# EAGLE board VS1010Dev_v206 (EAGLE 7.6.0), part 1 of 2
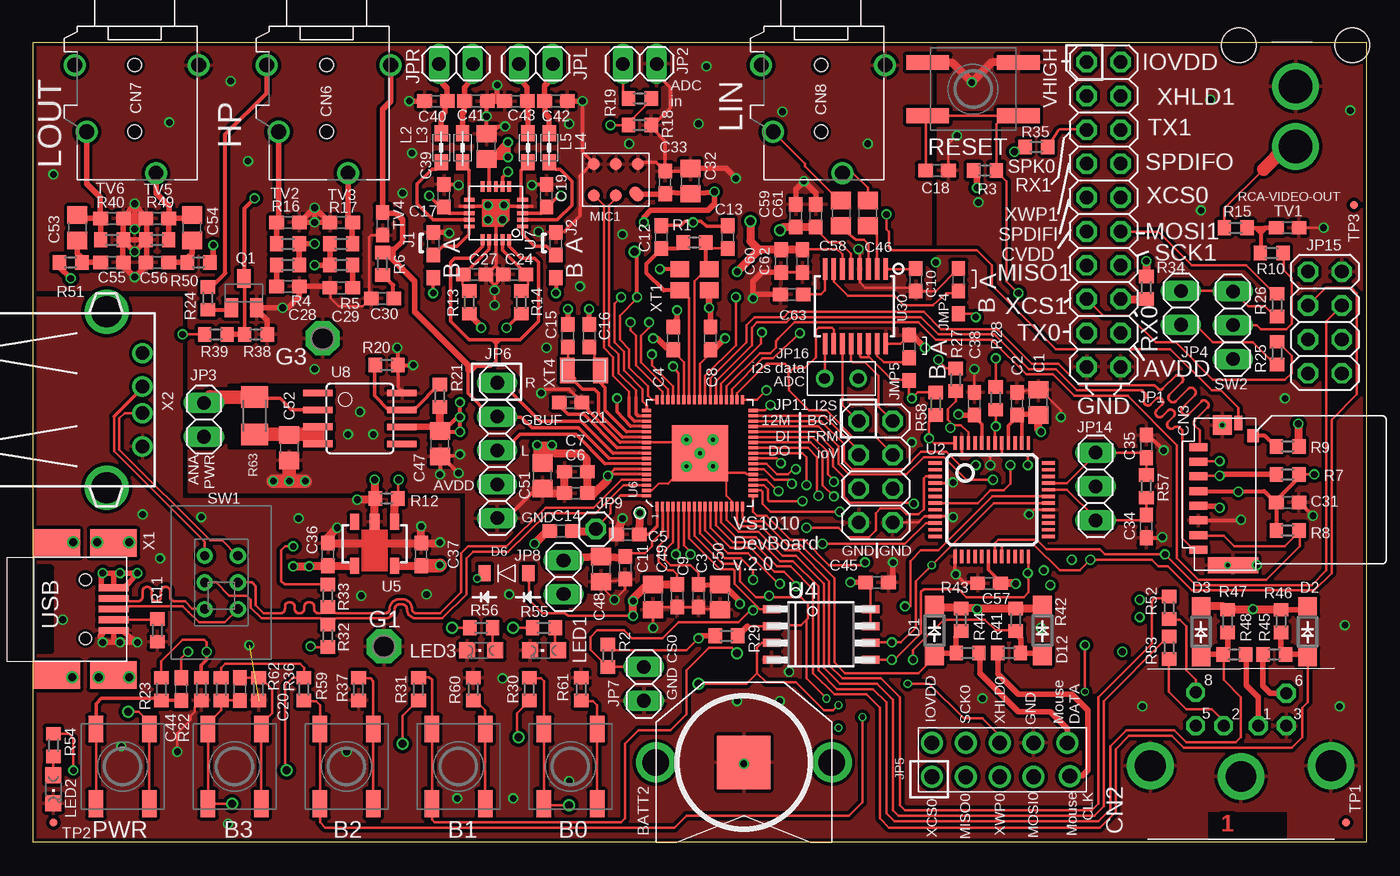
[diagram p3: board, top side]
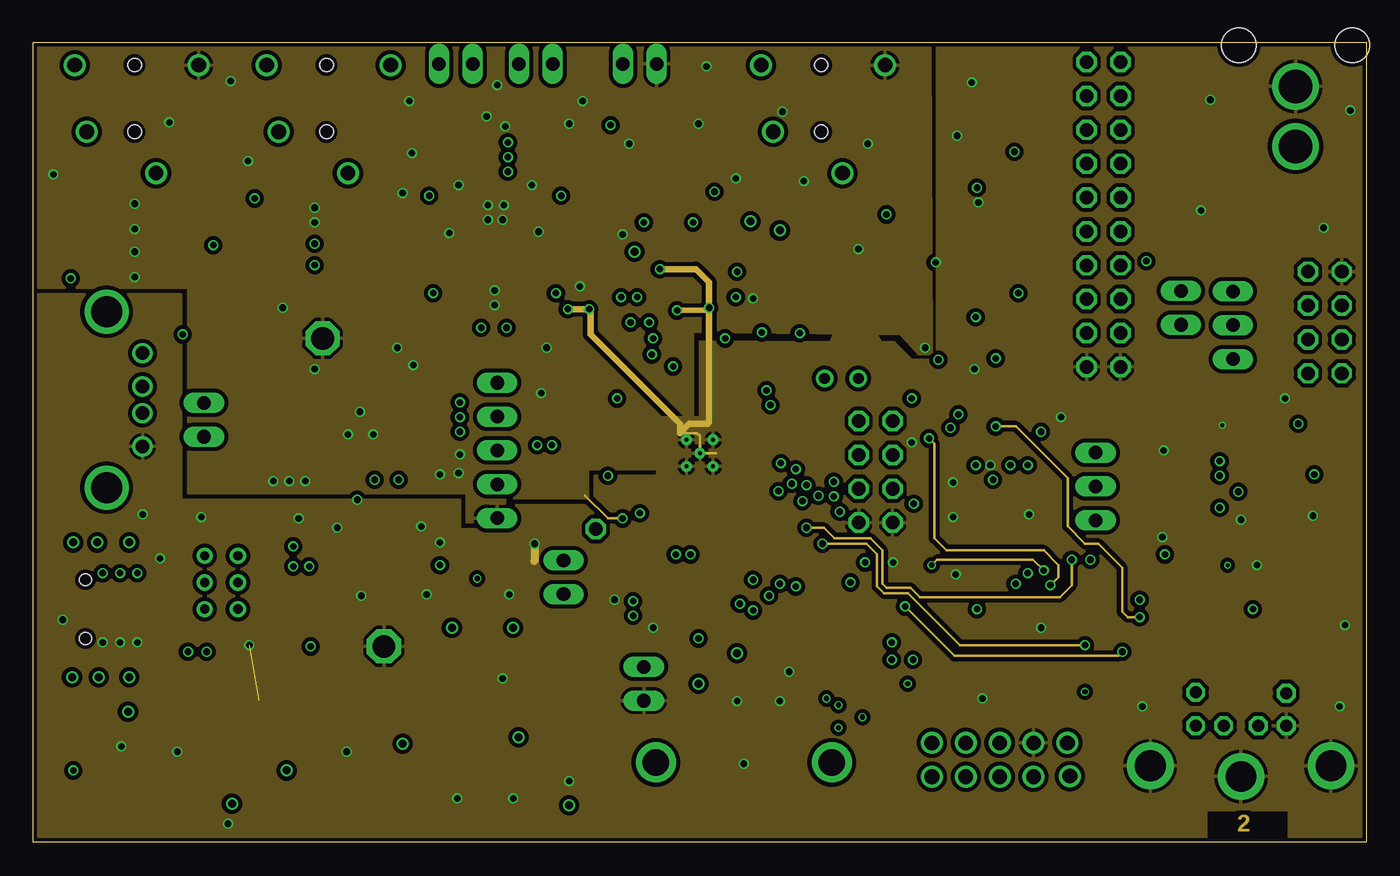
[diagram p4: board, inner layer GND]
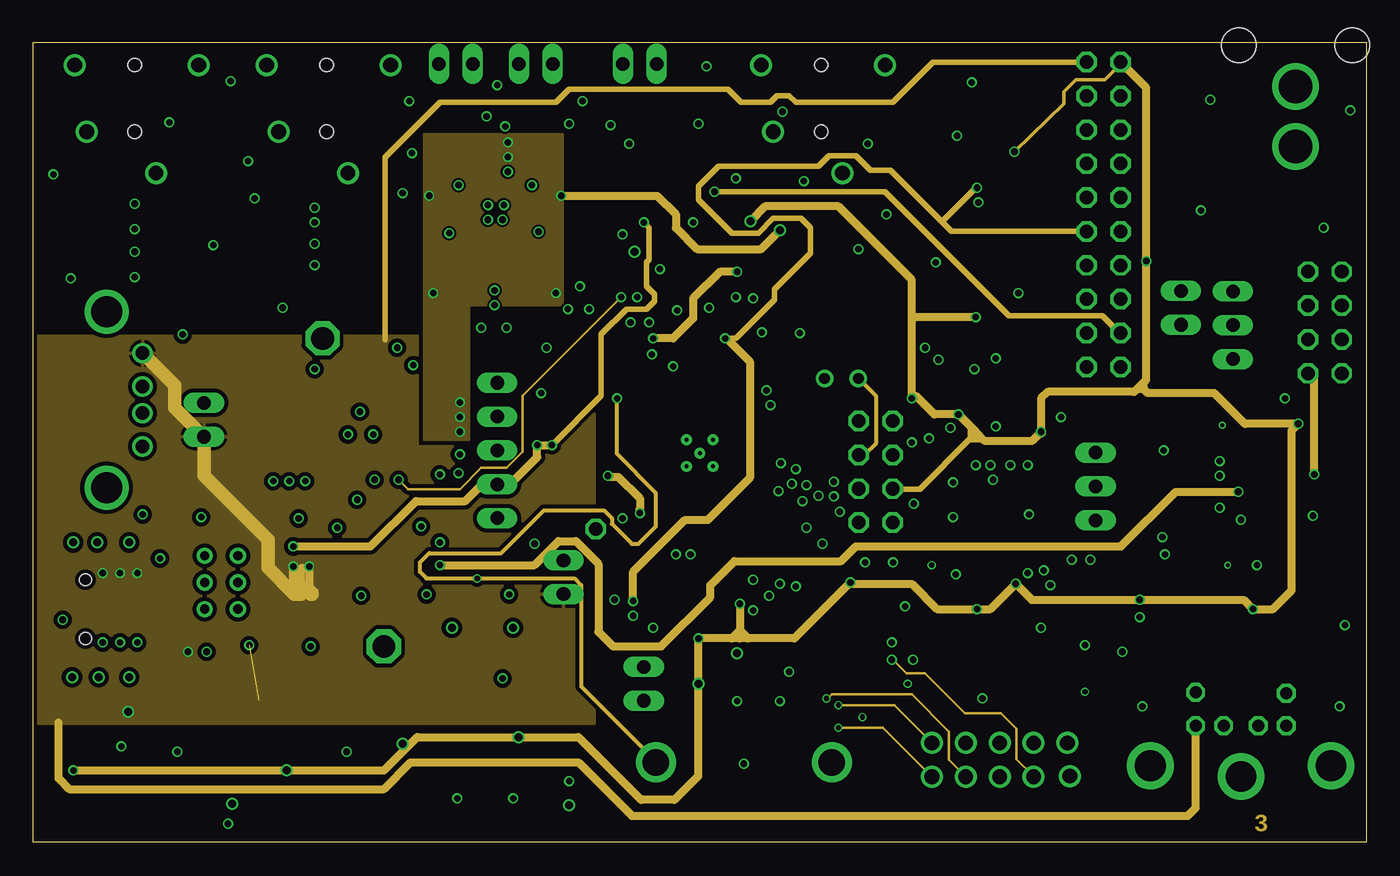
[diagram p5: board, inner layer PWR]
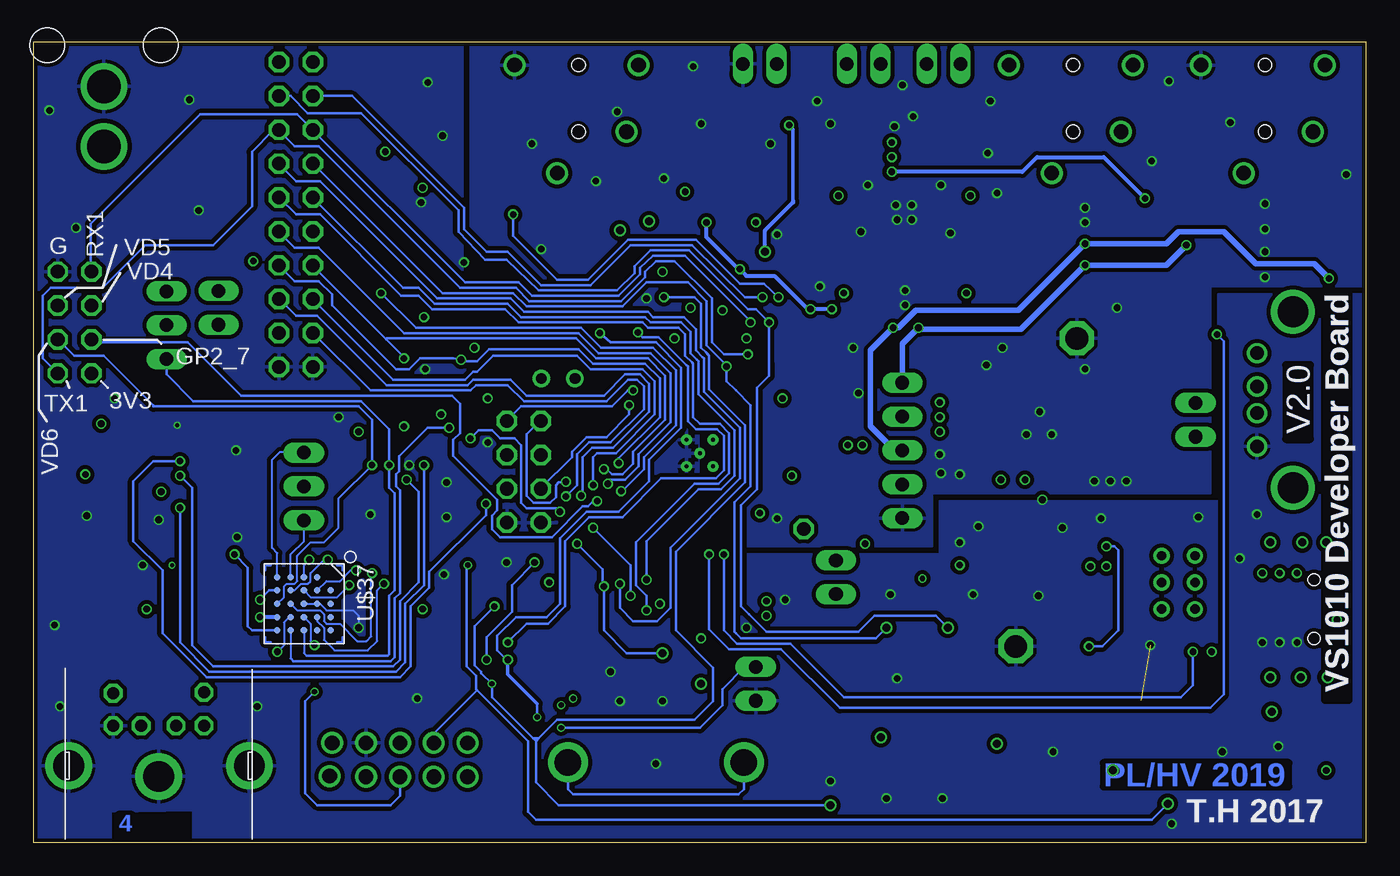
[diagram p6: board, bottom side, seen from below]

Size 100 x 60 mm. Coordinates in mm from the lower left corner, seen from the top.
Outline: 100,0 0,0 0,60 100,60 100,0
Copper layers ((1*2+3*16)): Top 0.035mm / dielectric 0.12mm / GND 0.0175mm / dielectric 1.2mm / PWR 0.035mm / dielectric 0.2mm / Bottom 0.035mm
Design rules "4L_Smart_prototyping_Eagle Rule *": minimum track width 6mil, minimum drill 0.3mm, track to track 6mil, track to pad 6mil, pad to pad 6mil, via to via 6mil, smd to smd 0mil, copper to edge 6mil, drill to drill 12mil, minimum pad ring 10mil, minimum via ring 4mil, stop-mask expansion 2mil, vias tented up to drill 25mil, thermal gap 10mil
tRestrict: area 48.5,25.6 to 53.6,32.8; area 33.1,45.6 to 36.3,48.8

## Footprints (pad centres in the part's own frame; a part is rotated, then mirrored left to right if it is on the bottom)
SW_EVQ_MINI = smd 2 x 1.1: A -2.8,2; A1 2.8,2; B -2.8,-2; B1 2.8,-2
KS2997 = smd 4 x 4: NEG 0,0 | drill 2: P1 -6.6,0; P2 6.6,0
C0805 = smd 1.3 x 1.5: 1 -0.95,0; 2 0.95,0
C0603 = smd 1.1 x 1: 1 -0.85,0; 2 0.85,0
M_DIN6 = drill 0.9 pad 1.422 octagon: 1 -1.3,-3.75; 2 1.3,-3.75; 3 -3.4,-3.75; 5 3.4,-3.75; 6 -3.4,-6.2; 8 3.4,-6.25 | drill 2.3 pad 3.5: SH1 6.8,-0.75; SH2 0,0.05; SH3 -6.75,-0.75
MSSN09-A0-3000 = smd 0.6 x 1.35: 1 3.85,0.1; 2 2.75,0.1; 3 1.65,0.1; 4 0.55,0.1; 5 -0.55,0.1; 6 -1.65,0.1; 7 -2.75,0.1; 8 -3.85,0.1 | smd 1.2 x 3.79: 9 -5,-2.5 | smd 1.45 x 1.4: 10 5.5,-1.7 | smd 1.1 x 0.6: 11 5.65,-2.9 | smd 0.95 x 0.85: 12 4.7,-4
SJ-43514 = drill 1.1: 1 8.1,1.6; 4 5,-3.6; 5 0,4.8; 6 0,-4.5 | hole 1: 0,0; 5,0
SOD123 = smd 1.4 x 1.4: A 1.9,0; C -1.9,0
SOD-123 = smd 0.914 x 1.219: ANODE -1.638,0; CATHODE 1.638,0
P1-17 = drill 1.702 pad 2.54 octagon: TP 0,0
0603X2 = smd 1.1 x 1: 1 -0.85,0; 2 0.85,0; 3 2.55,0
2X10 = drill 1.016 octagon: 1 -11.43,-1.27; 2 -11.43,1.27; 3 -8.89,-1.27; 4 -8.89,1.27; 5 -6.35,-1.27; 6 -6.35,1.27; 7 -3.81,-1.27; 8 -3.81,1.27; 9 -1.27,-1.27; 10 -1.27,1.27; 11 1.27,-1.27; 12 1.27,1.27; 13 3.81,-1.27; 14 3.81,1.27; 15 6.35,-1.27; 16 6.35,1.27; 17 8.89,-1.27; 18 8.89,1.27; 19 11.43,-1.27; 20 11.43,1.27
1X02 = drill 1.016 long: 1 -1.27,0; 2 1.27,0
2X5_2.54MM_CON = drill 1.1: 1 -5.08,-1.27; 2 -5.08,1.27; 3 -2.54,-1.27; 4 -2.54,1.27; 5 0,-1.27; 6 0,1.27; 7 2.54,-1.27; 8 2.54,1.27; 9 5.27,-1.22; 10 5.08,1.27
1X05 = drill 1.016 long: 1 -5.08,0; 2 -2.54,0; 3 0,0; 4 2.54,0; 5 5.08,0
1X01 = drill 1.016 octagon: 1 0,0
2X04 = drill 1.016 octagon: 1 -3.81,-1.27; 2 -3.81,1.27; 3 -1.27,-1.27; 4 -1.27,1.27; 5 1.27,-1.27; 6 1.27,1.27; 7 3.81,-1.27; 8 3.81,1.27
1X03 = drill 1.016 long: 1 -2.54,0; 2 0,0; 3 2.54,0
2X1_2.54MM_CON_THROUGH = drill 0.8: P$1 0,0; P$2 2.54,0
0805 = smd 1.2 x 1: 1 -1.1,0; 2 1.1,0
CHIPLED_0805 = smd 1.2 x 1.2: A 0,-1.05; C 0,1.05
MIC_MEMS_CMM-4737DT = smd 0.91 x 0.91: 1 -1.17,1.65; 2 -1.17,0; 3 -1.17,-1.65; 4 1.17,-1.65; 5 1.17,0 | smd 1.2 x 0.91 rotated 45: 6 1.07,1.55
SOT23-BEC = smd 1 x 1.4: B -0.95,-1.1; C 0,1.1; E 0.95,-1.1
R0603 = smd 1 x 1.1: 1 -0.85,0; 2 0.85,0
M1206 = smd 1.6 x 2: 1 -1.4,0; 2 1.4,0
1X1_RCA_CON_RCJ-044 = drill 2.5: 1 -4,0; 2 -8.5,0 | hole 2.6: -0.9,4.25; -0.9,-4.25
SW_EVQ = smd 3.2 x 1.1: A -3.4,2; A1 3.4,2; B -3.4,-2; B1 3.4,-2
SW_ALPS_SSSS922500 = drill 0.7: 1 -2,-1.25; 2 0,-1.25; 3 2,-1.25; 4 -2,1.25; 5 0,1.25; 6 2,1.25
TP06R = smd 0.6 x 0.6: TP 0,0
0603 = smd 1.1 x 1: 1 -0.85,0; 2 0.85,0
LQFP48 = smd 0.25 x 1: 1 -2.75,-4.25; 2 -2.25,-4.25; 3 -1.75,-4.25; 4 -1.25,-4.25; 5 -0.75,-4.25; 6 -0.25,-4.25; 7 0.25,-4.25; 8 0.75,-4.25; 9 1.25,-4.25; 10 1.75,-4.25; 11 2.25,-4.25; 12 2.75,-4.25; 25 2.75,4.25; 26 2.25,4.25; 27 1.75,4.25; 28 1.25,4.25; 29 0.75,4.25; 30 0.25,4.25; 31 -0.25,4.25; 32 -0.75,4.25; 33 -1.25,4.25; 34 -1.75,4.25; 35 -2.25,4.25; 36 -2.75,4.25 | smd 1 x 0.25: 13 4.25,-2.75; 14 4.25,-2.25; 15 4.25,-1.75; 16 4.25,-1.25; 17 4.25,-0.75; 18 4.25,-0.25; 19 4.25,0.25; 20 4.25,0.75; 21 4.25,1.25; 22 4.25,1.75; 23 4.25,2.25; 24 4.25,2.75; 37 -4.25,2.75; 38 -4.25,2.25; 39 -4.25,1.75; 40 -4.25,1.25; 41 -4.25,0.75; 42 -4.25,0.25; 43 -4.25,-0.25; 44 -4.25,-0.75; 45 -4.25,-1.25; 46 -4.25,-1.75; 47 -4.25,-2.25; 48 -4.25,-2.75
SO8-SHORT = smd 1.3 x 0.6: 1 -3.913,1.905; 2 -3.913,0.635; 3 -3.913,-0.635; 4 -3.913,-1.905; 5 3.513,-1.905; 6 3.513,-0.635; 7 3.513,0.635; 8 3.513,1.905
SOT89-5 = smd 0.68 x 1.2: 1 -1.5,-1.65; 3 1.5,-1.65; 4 1.5,1.65; 5 -1.5,1.65 | smd 0.76 x 1.2: 2 0,-1.65
QFN68 = smd 0.7 x 0.23: 1 -4,3.2; 2 -4,2.8; 3 -4,2.4; 4 -4,2; 5 -4,1.6; 6 -4,1.2; 7 -4,0.8; 8 -4,0.4; 9 -4,0; 10 -4,-0.4; 11 -4,-0.8; 12 -4,-1.2; 13 -4,-1.6; 14 -4,-2; 15 -4,-2.4; 16 -4,-2.8; 17 -4,-3.2; 35 4,-3.2; 36 4,-2.8; 37 4,-2.4; 38 4,-2; 39 4,-1.6; 40 4,-1.2; 41 4,-0.8; 42 4,-0.4; 43 4,0; 44 4,0.4; 45 4,0.8; 46 4,1.2; 47 4,1.6; 48 4,2; 49 4,2.4; 50 4,2.8; 51 4,3.2 | smd 0.23 x 0.7: 18 -3.2,-4; 19 -2.8,-4; 20 -2.4,-4; 21 -2,-4; 22 -1.6,-4; 23 -1.2,-4; 24 -0.8,-4; 25 -0.4,-4; 26 0,-4; 27 0.4,-4; 28 0.8,-4; 29 1.2,-4; 30 1.6,-4; 31 2,-4; 32 2.4,-4; 33 2.8,-4; 34 3.2,-4; 52 3.2,4; 53 2.8,4; 54 2.4,4; 55 2,4; 56 1.6,4; 57 1.2,4; 58 0.8,4; 59 0.4,4; 60 0,4; 61 -0.4,4; 62 -0.8,4; 63 -1.2,4; 64 -1.6,4; 65 -2,4; 66 -2.4,4; 67 -2.8,4; 68 -3.2,4 | smd 4.2 x 4.2: GNDPAD 0,0 | drill 0.3: P$1 -1,1; P$2 1,1; P$3 1,-1; P$4 -1,-1; P$5 0,0
QFN20 = smd 0.8 x 0.28: 1 -2,1; 2 -2,0.5; 3 -2,0; 4 -2,-0.5; 5 -2,-1; 11 2,-1; 12 2,-0.5; 13 2,0; 14 2,0.5; 15 2,1 | smd 0.28 x 0.8: 6 -1,-2; 7 -0.5,-2; 8 0,-2; 9 0.5,-2; 10 1,-2; 16 1,2; 17 0.5,2; 18 0,2; 19 -0.5,2; 20 -1,2
SOIC8 = smd 0.5 x 2.2: 1 -1.905,-3.354; 2 -0.645,-3.354; 3 0.625,-3.354; 4 1.895,-3.354; 5 1.905,2.954; 6 0.635,2.954; 7 -0.635,2.954; 8 -1.905,2.954
TSSOP16 = smd 1.6 x 0.35: 1 -2.9,2.45; 2 -2.9,1.8; 3 -2.9,1.15; 4 -2.9,0.5; 5 -2.9,-0.15; 6 -2.9,-0.8; 7 -2.9,-1.45; 8 -2.9,-2.1; 9 2.7,-2.1; 10 2.7,-1.45; 11 2.7,-0.8; 12 2.7,-0.15; 13 2.7,0.5; 14 2.7,1.15; 15 2.7,1.8; 16 2.7,2.45
BGA24_5X5 = smd 0.5 x 0.5: A2 1,0; A3 2,0; A4 3,0; A5 4,0; B1 0,-1; B2 1,-1; B3 2,-1; B4 3,-1; B5 4,-1; C1 0,-2; C2 1,-2; C3 2,-2; C4 3,-2; C5 4,-2; D1 0,-3; D2 1,-3; D3 2,-3; D4 3,-3; D5 4,-3; E1 0,-4; E2 1,-4; E3 2,-4; E4 3,-4; E5 4,-4
MINI_USB_MOLEX-B = smd 2.25 x 0.5: 1 7.915,1.6; 2 7.915,0.8; 3 7.915,0; 4 7.915,-0.8; 5 7.915,-1.6 | smd 3.5 x 2.05: P$6 7.915,4.95; P$7 7.915,-4.95; P$8 3.665,4.95; P$9 3.665,-4.95 | hole 0.9: 5.815,2.2; 5.815,-2.2
USB-S = drill 1: 1 -3.5,12.99; 2 -1,12.99; 3 1,12.99; 4 3.5,12.99 | drill 2.3: P$1 -6.6,10.3; P$2 6.6,10.3
NX3225GA = smd 1.4 x 1.2: 1 -1.1,-0.8; 2 1.1,-0.8; 3 1.1,0.8; 4 -1.1,0.8
CRYSTAL_1206 = smd 1.1 x 1.9: 1 -1.25,0; 2 1.25,0

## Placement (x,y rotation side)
B0  [SW_EVQ_MINI]  40.3,5.7 90 top
B1  [SW_EVQ_MINI]  31.9,5.7 90 top
B2  [SW_EVQ_MINI]  23.5,5.7 90 top
B3  [SW_EVQ_MINI]  15.1,5.7 90 top
BATT2  1.5V LR(SR)44  [KS2997]  53.3,6 180 top
C1  10u  [C0805]  75.4,33 90 top
C2  100n  [C0603]  73.8,32.9 90 top
C3  100n  [C0603]  49.9,18.5 270 top
C4  100n  [C0603]  48,37.8 90 top
C5  100n  [C0603]  44.6,23.1 180 top
C6  100n  [C0603]  40.7,26.2 180 top
C7  100n  [C0603]  40.7,27.8 180 top
C8  100n  [C0603]  50.8,37.8 90 top
C9  100n  [C0603]  48.3,18.5 270 top
C10  470n  [C0603]  66.2,42.2 270 top
C11  100n  [C0603]  44.4,20.6 270 top
C12  4.7p  [C0603]  47.1,45.4 270 top
C13  4.7p  [C0603]  52.1,45.4 270 top
C14  1u  [C0603]  39.59,23.36 180 top
C15  10P  [C0603]  40.1,38 270 top
C16  10P  [C0603]  41.7,38 270 top
C17  100n  [C0603]  30.8,48.5 90 top
C18  1u  [C0603]  67.8,50.4 0 top
C19  100n  [C0603]  38.5,48.5 90 top
C20  100n  [C0603]  15.5,11.5 90 top
C21  1u  [C0603]  40.3,33 0 top
C24  4n7/NP0  [C0603]  36.1,42.6 180 top
C27  4n7/NP0  [C0603]  33.1,42.6 0 top
C28  10n  [C0603]  19.1,41.7 0 top
C29  10n  [C0603]  23.1,41.6 180 top
C30  47n  [C0603]  26.2,40.8 180 top
C31  1u  [C0603]  94.1,25.5 0 top
C32  10u  [C0805]  49.3,49.6 270 top
C33  100n  [C0603]  47.4,49.5 90 top
C34  20P  [C0603]  83.5,23.7 90 top
C35  20P  [C0603]  83.5,29.7 270 top
C36  1u  [C0603]  22.1,21.6 90 top
C37  1u  [C0603]  29.1,21.6 90 top
C38  100n  [C0603]  70.6,32.9 90 top
C39  10u  [C0805]  34,52.2 90 top
C40  1n  [C0603]  30.2,55.6 180 top
C41  1n  [C0603]  33.2,55.6 0 top
C42  1n  [C0603]  39.2,55.6 0 top
C43  1n  [C0603]  36.2,55.6 180 top
C44  dnc  [C0603]  11.1,11.5 90 top
C45  100n  [C0603]  63.3,19.5 0 top
C46  10u  [C0805]  62.6,47.2 270 top
C47  10u  [C0805]  30.5,29.9 90 top
C48  10u  [C0805]  42.6,20.5 270 top
C49  10u  [C0805]  46.5,18.4 270 top
C50  10u  [C0805]  51.5,18.4 270 top
C51  10u  [C0805]  38.2,27.5 270 top
C52  10u  [C0805]  19.2,29.6 270 top
C53  10u  [C0805]  3.3,46.1 90 top
C54  10u  [C0805]  11.9,46.1 90 top
C55  3n3/NP0  [C0603]  5.9,43.5 0 top
C56  3n3/NP0  [C0603]  9.3,43.5 180 top
C57  100n  [C0603]  71.7,19.44 180 top
C58  10u  [C0805]  60.6,47.2 270 top
C59  10u  [C0603]  57.2,47 270 top
C60  10u  [C0603]  56.1,43.6 270 top
C61  100n  [C0603]  58.7,47 270 top
C62  100n  [C0603]  57.7,43.6 270 top
C63  1u  [C0603]  56.9,41.1 180 top
CN2  [M_DIN6]  90.6,5 180 top
CN3  CON-USD-TOMIN  [MSSN09-A0-3000]  87.5,25.8 90 top
CN6  SJ-43514  [SJ-43514]  22,58.3 270 top
CN7  SJ-43514  [SJ-43514]  7.6,58.3 270 top
CN8  SJ-43514  [SJ-43514]  59.1,58.3 270 top
D1  SD103AW  [SOD123]  67.6,15.9 270 top
D2  SD103AW  [SOD123]  95.6,15.8 270 top
D3  SD103AW  [SOD123]  87.6,15.8 270 top
D6  MBR0520  [SOD-123]  35.5,20.2 180 top
D12  SD103AW  [SOD123]  75.7,15.9 270 top
G1  TPPAD1-17  [P1-17]  26.3,14.7 0 top
G3  TPPAD1-17  [P1-17]  21.7,37.8 0 top
J1  100K  [0603X2]  30,44.9 270 top
J2  100K  [0603X2]  39.2,44.9 270 top
JMP4  0R-JMP  [0603X2]  69.4,42.2 270 top
JMP5  0R-JMP  [0603X2]  65.7,37.2 270 top
JP1  [2X10]  80.3,47.1 270 top
JP2  [1X02]  45.5,58.4 180 top
JP3  [1X02]  12.8,31.7 270 top
JP4  [1X02]  86.1,40.1 270 top
JP5  spi0/mouse  [2X5_2.54MM_CON]  72.5,6.2 0 top
JP6  [1X05]  34.8,29.4 270 top
JP7  [1X02]  45.8,11.9 90 top
JP8  [1X02]  39.78,19.89 270 top
JP9  [1X01]  42.2,23.5 0 top
JP11  [2X04]  63.2,27.8 270 top
JP14  SMC-1-03-1-GT  [1X03]  79.7,26.7 270 top
JP15  [2X04]  96.9,39 270 top
JP16  [2X1_2.54MM_CON_THROUGH]  61.9,34.8 180 top
JPL  SPKL  [1X02]  37.7,58.4 180 top
JPR  SPKR  [1X02]  31.7,58.4 0 top
L2  [0805]  30.6,52.1 90 top
L3  [0805]  32.2,52.1 90 top
L4  [0805]  38.7,52.1 90 top
L5  [0805]  37.1,52.1 90 top
LED1  GREEN  [CHIPLED_0805]  38.3,14.4 90 top
LED2  GREEN  [CHIPLED_0805]  1.5,4 180 top
LED3  RED  [CHIPLED_0805]  33.6,14.4 90 top
MIC1  cmm-4737DT-26186-TR  [MIC_MEMS_CMM-4737DT]  43.7,49.7 270 top
PWR  [SW_EVQ_MINI]  6.7,5.7 90 top
Q1  BC850  [SOT23-BEC]  15.8,41.2 0 top
R1  470k  [R0603]  49.6,45 0 top
R2  100k  [R0603]  43.1,14 270 top
R3  100k  [R0603]  71.4,50.4 0 top
R4  20R  [R0603]  19.1,43.3 180 top
R5  20R  [R0603]  23.1,43.3 0 top
R6  10R  [R0603]  26.2,43.4 270 top
R7  11k  [R0603]  94.1,27.6 180 top
R8  11k  [R0603]  94.1,23.4 0 top
R9  11k  [R0603]  94.1,29.7 180 top
R10  22R  [R0603]  92.9,44.2 180 top
R11  100k  [R0603]  9.3,15.9 270 top
R12  100k  [R0603]  26.5,25.8 180 top
R13  1k  [R0603]  32.7,40.5 270 top
R14  1k  [R0603]  36.6,40.5 270 top
R15  22R  [R0603]  90.2,46.1 180 top
R16  10R  [R0603]  19.1,44.9 180 top
R17  10R  [R0603]  23.1,44.9 0 top
R18  2k  [R0603]  45.5,53.8 0 top
R19  18k  [R0603]  45.5,55.8 0 top
R20  11k  [R0603]  26.5,35.8 180 top
R21  51k  [R0603]  30.5,33.5 270 top
R22  100k  [R0603]  12.6,11.5 90 top
R23  51k  [R0603]  9.6,11.5 90 top
R24  100k  [R0603]  13.1,40.8 270 top
R25  100R  [R0603]  93.3,36.7 90 top
R26  100R  [R0603]  93.3,40.3 90 top
R27  11k  [R0603]  69.2,34.7 90 top
R28  11k  [R0603]  72.2,33.3 270 top
R29  100k  [R0603]  52,15.5 0 top
R30  100k  [R0603]  37.2,11.5 270 top
R31  100k  [R0603]  28.9,11.5 270 top
R32  470k  [R0603]  22.1,15.5 90 top
R33  470k  [R0603]  22.1,18.5 270 top
R34  100k  [R0603]  83.5,41.6 90 top
R35  100k  [R0603]  75.25,52.17 180 top
R36  11k  [R0603]  16.9,11.5 270 top
R37  11k  [R0603]  24.4,11.5 270 top
R38  51k  [R0603]  16.7,38.1 0 top
R39  11k  [R0603]  13.7,38.1 0 top
R40  100k  [R0603]  5.9,45.2 0 top
R41  330R  [R0603]  73.2,14.2 0 top
R42  2k  [R0603]  73.7,16.7 270 top
R43  2k  [R0603]  69.6,16.7 270 top
R44  330R  [R0603]  70.1,14.2 0 top
R45  330R  [R0603]  93.1,14.1 180 top
R46  2k  [R0603]  93.6,16.6 270 top
R47  2k  [R0603]  89.6,16.6 270 top
R48  330R  [R0603]  90.1,14.1 180 top
R49  100k  [R0603]  9.3,45.2 180 top
R50  470R  [R0603]  12.4,43.5 180 top
R51  470R  [R0603]  2.8,43.5 0 top
R52  11k  [R0603]  85.2,17.6 90 top
R53  11k  [R0603]  85.2,14.6 90 top
R54  330R  [R0603]  1.5,7.3 270 top
R55  330R  [R0603]  38.3,16.1 0 top
R56  330R  [R0603]  33.6,16.1 0 top
R57  470k  [R0603]  83.5,26.7 270 top
R58  11k  [R0603]  67.7,32.9 270 top
R59  100k  [R0603]  20.3,11.5 90 top
R60  11k  [R0603]  33,11.5 90 top
R61  11k  [R0603]  41.1,11.5 90 top
R62  100k  [R0603]  14.1,11.5 90 top
R63  0  [M1206]  16.6,32 90 top
RCA-VIDEO-OUT  1X1_RCA_CON_RCJ-044  [1X1_RCA_CON_RCJ-044]  94.7,60.7 90 top
RESET  [SW_EVQ]  70.5,56.5 0 top
SW1  SSSS922500  [SW_ALPS_SSSS922500]  14.1,19.5 90 top
SW2  [1X03]  90,38.8 90 top
TP1  TPSTP06R  [TP06R]  98.5,1.5 0 top
TP2  TPSTP06R  [TP06R]  1.5,1.5 0 top
TP3  TPSTP06R  [TP06R]  99.1,47.8 0 top
TV1  CG0603MLA-5.5ME  [0603]  94.1,46.1 0 top
TV2  CG0603MLA-5.5ME  [0603]  19.1,46.5 0 top
TV3  CG0603MLA-5.5ME  [0603]  23.1,46.5 180 top
TV4  CG0603MLA-5.5ME  [0603]  26.2,46.4 270 top
TV5  CG0603MLA-5.5ME  [0603]  9.3,46.8 180 top
TV6  CG0603MLA-5.5ME  [0603]  5.9,46.8 0 top
U2  VS23S010C48-L  [LQFP48]  71.9,25.7 270 top
U4  25LCXXXXSOS  [SO8-SHORT]  59.3,15.6 0 top
U5  AP7361C-33Y5-13  [SOT89-5]  25.6,22.4 180 top
U6  VS1010-68_NEW2Q  [QFN68]  50,29.2 90 top
U7  CP2122  [QFN20]  34.7,47.2 180 top
U8  AP2318M-ADJTRG1  [SOIC8]  24.7,31.8 270 top
U30  AK5720  [TSSOP16]  61.5,40.1 270 top
U$37  VS23S040D-B  [BGA24_5X5]  77.7,19.9 270 bottom
X1  [MINI_USB_MOLEX-B]  -1.9,17.5 0 top
X2  [USB-S]  -4.8,33.2 270 top
XT1  NX3225GA  [NX3225GA]  49.6,42.2 0 top
XT4  32.768KHz/12pF  [CRYSTAL_1206]  41.3,35.4 0 top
